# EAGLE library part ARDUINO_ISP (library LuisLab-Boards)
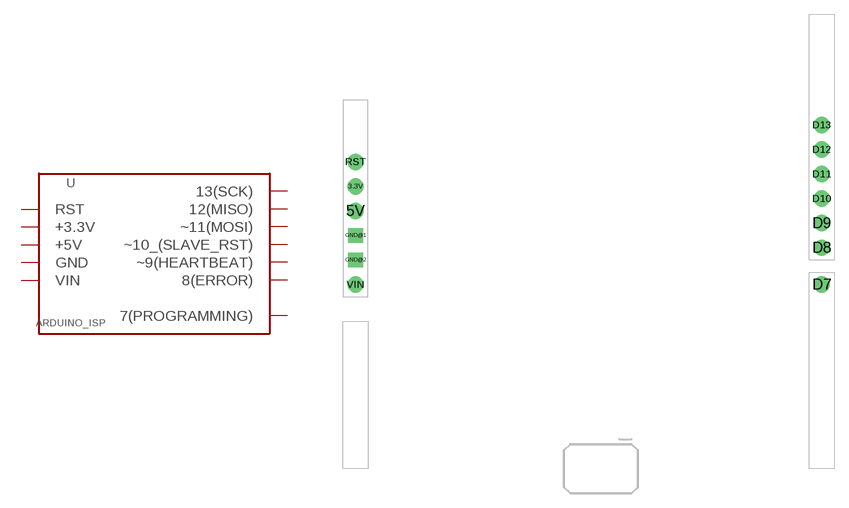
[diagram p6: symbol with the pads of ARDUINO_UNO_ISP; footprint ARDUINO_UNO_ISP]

Designator prefix -

## ARDUINO_ISP_UNO  [ARDUINO_UNO_ISP]
3.3V  +3.3V
5V  +5V
D7  7(PROGRAMMING)
D8  8(ERROR)
D9  ~9(HEARTBEAT)
D10  ~10_(SLAVE_RST)
D11  ~11(MOSI)
D12  12(MISO)
D13  13(SCK)
GND@1  GND
GND@2  GND
RST  RST
VIN  VIN

## Footprint ARDUINO_UNO_ISP (pad centres in mm)
drill 1.016 pad 1.7: 3.3V -24.13,1.27; 5V -24.13,-1.27; D7 24.13,-8.89; D8 24.13,-5.08; D9 24.13,-2.54; D10 24.13,0; D11 24.13,2.54; D12 24.13,5.08; D13 24.13,7.62; RST -24.13,3.81; VIN -24.13,-8.89
drill 1.016 pad 1.5 square: GND@1 -24.13,-3.81; GND@2 -24.13,-6.35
